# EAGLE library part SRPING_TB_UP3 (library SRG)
Spring loaded Terminal block 4UCON 0.10 pitch straight (wire goes in top) 2 amps 20-26 AWG Adafruit: P/N 1081
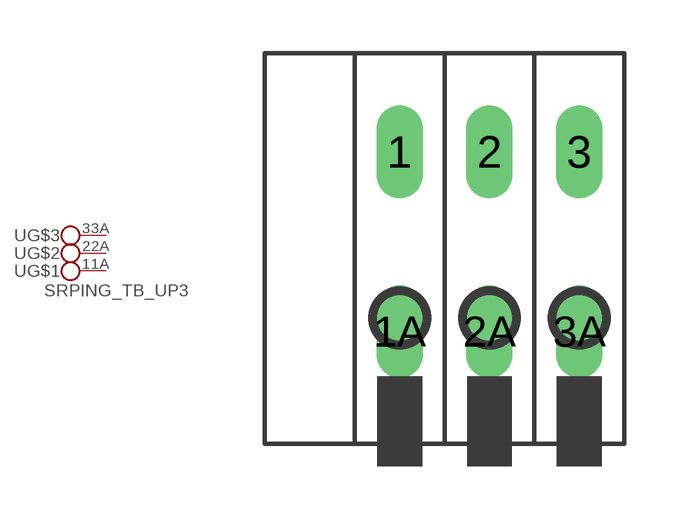
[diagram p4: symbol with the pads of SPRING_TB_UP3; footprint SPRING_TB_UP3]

Designator prefix -; gates G$1=KL2V G$2=KL2 G$3=KL2

## SRPING_TB_UP3  [SPRING_TB_UP3]
1  G$1:1  pas
1A  G$1:2  pas
2  G$2:1  pas
2A  G$2:2  pas
3  G$3:1  pas
3A  G$3:2  pas

## Footprint SPRING_TB_UP3 (pad centres in mm)
Spring Loaded Terminal Block 4UCON 0.10 pitch straight (wire goes in top) 2 amps 20-26 AWG Adafruit: P/N 1081 Terminal block comes with 3 terminals, but the are modular so you can add or remove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
drill 0.8 long: 1 -2.54,2.54; 1A -2.54,-2.54; 2 0,2.54; 2A 0,-2.54; 3 2.54,2.54; 3A 2.54,-2.54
